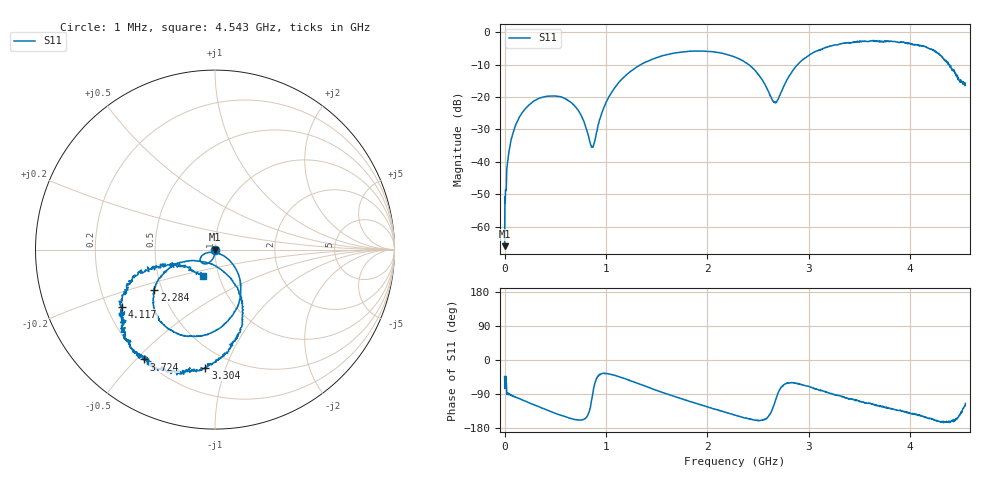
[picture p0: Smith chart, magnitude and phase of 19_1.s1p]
# HZ S RI R 50
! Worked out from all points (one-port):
!   1515 points, 1 MHz to 4.543 GHz, reference 50 ohm
!   lowest |S11| = -66.1 dB at 1 MHz (marker M1), VSWR 1.00, Z = 50 - j0.0343 ohm
!   |S11| at or under -10 dB: start of sweep to 1.342 GHz; 2.408 GHz to 2.889 GHz (481.1 MHz wide, 18.2 % of centre); 4.383 GHz to end of sweep
!   S11 on the Smith chart (normalised r, x): 1 MHz: 1.00, -0.00; 2.284 GHz: 0.45, -0.25; 3.304 GHz: 0.37, -0.85; 3.724 GHz: 0.20, -0.53; 4.117 GHz: 0.26, -0.26; 4.543 GHz: 0.84, -0.26
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1000000  0.000361 -0.000343
2.5e7  -0.000194 -0.00834
4.3e7  0.000312 -0.0142
7.9e7  -0.00181 -0.0262
1.27e8  -0.00697 -0.0414
3.16e8  -0.0469 -0.0786
5.71e8  -0.0828 -0.0537
7.33e8  -0.0557 -0.0221
8.68e8  -0.000792 -0.0169
9.91e8  0.0615 -0.0436
1.138e9  0.1242 -0.1244
1.372e9  0.1279 -0.3091
1.705e9  -0.0736 -0.4805
2.041e9  -0.3021 -0.4007
2.272e9  -0.3413 -0.2339
2.284e9  -0.338 -0.226
2.476e9  -0.2339 -0.0926
2.662e9  -0.0344 -0.0744
2.842e9  0.1266 -0.2236
3.034e9  0.1403 -0.4548
3.304e9  -0.0539 -0.6577
3.409e9  -0.1426 -0.6653
3.724e9  -0.3942 -0.6121
3.976e9  -0.5009 -0.4342
4.117e9  -0.518 -0.3179
4.351e9  -0.3499 -0.1059
4.489e9  -0.1401 -0.0972
4.543e9  -0.0683 -0.1485
